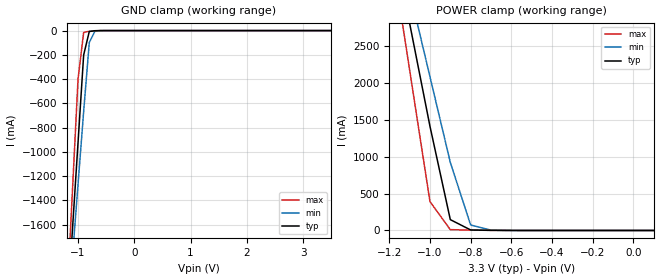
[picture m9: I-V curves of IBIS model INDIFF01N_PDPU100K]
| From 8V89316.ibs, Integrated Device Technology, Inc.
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[Model]   INDIFF01N_PDPU100K
Model_type   Input
Polarity   Non-Inverting
Vinl = 0.8V
Vinh = 2.0V
|   typ   min   max
C_comp   2pF   1.5pF   2.5pF
|   typ   min   max
[Voltage range]   3.3V   3.135V   3.465V
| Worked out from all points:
|   GND clamp passes 1 mA (typ) near -0.67 V on its own axis
|   POWER clamp passes 1 mA (typ) near -0.65 V on its own axis
[GND_clamp]
|Voltage   I (typ)   I (min)   I (max)
-3.3V     -17.55A    -15.11A    -21.66A
-1.2V     -2.37A     -2.47A     -2.252A
-1.1V     -1.646A    -1.868A    -1.326A
-1V       -923.3mA   -1.267A    -401.2mA
-900mV    -200.8mA   -666.1mA   -14.95mA
-800mV    -7.701mA   -98.82mA   -5.481mA
-700mV    -1.264mA   -4.706mA   -1.689mA
3.5V      1.998uA    5.205uA    371.3nA
[Power_clamp]
|Voltage   I (typ)   I (min)   I (max)
-3.3V     33.64A     28.92A     41.58A
-1.2V     4.209A     4.413A     3.966A
-1.1V     2.811A     3.249A     2.179A
-1V       1.414A     2.086A     391.8mA
-900mV    147.1mA    923.6mA    11.32mA
-800mV    6.896mA    74.43mA    4.727mA
-700mV    1.653mA    4.402mA    2.066mA
100mV     -997.6nA   -932.5nA   -1.061uA
